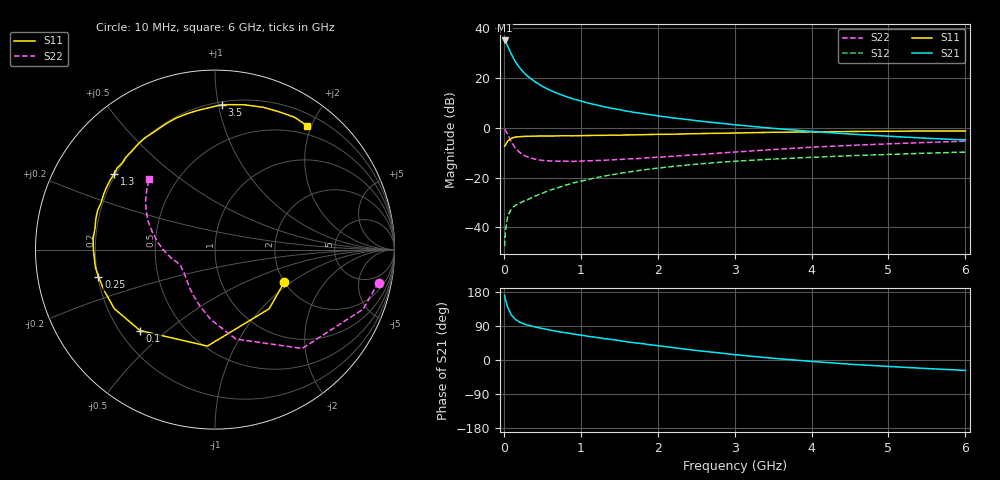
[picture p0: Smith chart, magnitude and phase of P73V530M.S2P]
! SIEMENS Small Signal Semiconductors
! BFP196
! Si NPN RF Bipolar Junction Transistor in SOT143
! VCE = 3.5 V  IC = 30 mA
! Common Emitter S-Parameters:  May  1996
# GHz  S  MA  R  50
!  f  S11  S21  S12  S22
! GHz  MAG  ANG  MAG  ANG  MAG  ANG  MAG  ANG
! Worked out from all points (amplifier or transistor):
!   36 points, 10 MHz to 6 GHz, reference 50 ohm
!   highest |S21| = 35.0 dB at 10 MHz (marker M1)
!   |S21| within 3 dB of that: start of sweep to 61.52 MHz
!   unconditionally stable (mu >= 1): 558.3 MHz to 3.966 GHz
!   at 250 MHz: K = 0.72, MSG = 26.0 dB, |S12| = -29.6 dB
!   at 1.4 GHz: K = 1.09, MAG = 11.5 dB, |S12| = -18.9 dB
!   at 6 GHz: K = 0.98, MSG = 2.4 dB, |S12| = -9.8 dB
!   lowest NFmin = 1.40 dB at 500 MHz
!   S11 on the Smith chart (normalised r, x): 10 MHz: 1.99, -0.89; 100 MHz: 0.28, -0.41; 250 MHz: 0.20, -0.11; 1.3 GHz: 0.19, +0.32; 3.5 GHz: 0.22, +1.03; 6 GHz: 0.37, +1.94
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0.01  0.4262 -25.4  56.22 170.6  0.0042 86.6  0.9293 -11.4
0.02  0.447 -47.5  53.38 160.6  0.0084 73.7  0.8897 -21.9
0.05  0.5392 -94.5  43.61 138.9  0.0169 58.6  0.7343 -48.6
0.1  0.6146 -132.8  29.32 118.2  0.0239 46.8  0.5121 -76.8
0.15  0.6505 -149.6  21.11 107.3  0.0277 44.2  0.3912 -93.3
0.2  0.6585 -159.8  16.38 100.6  0.0301 45.0  0.3256 -105.0
0.25  0.6666 -166.9  13.21 96.1  0.0332 47.1  0.2853 -114.4
0.3  0.6735 -171.5  11.12 92.7  0.0355 48.8  0.2625 -121.1
0.4  0.6771 -179.6  8.451 87.5  0.0421 52.2  0.2346 -131.5
0.5  0.6814 175.2  6.768 83.2  0.0485 54.5  0.2206 -138.9
0.6  0.6791 169.9  5.652 79.1  0.0559 56.3  0.2153 -144.1
0.7  0.6857 165.5  4.864 75.1  0.0622 57.2  0.2129 -148.0
0.9  0.6863 157.6  3.785 68.8  0.0776 57.4  0.211 -153.9
1.1  0.697 150.2  3.116 62.5  0.0918 56.8  0.2166 -157.7
1.3  0.7018 143.3  2.64 56.6  0.1066 55.3  0.2223 -161.3
1.7  0.7176 130.8  2.025 45.4  0.1344 51.1  0.2388 -167.3
2.2  0.7389 116.9  1.57 32.8  0.1674 44.7  0.2666 -174.4
3  0.7815 97.1  1.146 14.1  0.2125 33.9  0.3242 172.1
3.5  0.8086 87.2  0.97 4.6  0.2346 27.4  0.3644 164.0
4.5  0.8375 71.1  0.746 -11.1  0.2738 15.6  0.4414 150.3
5.5  0.8606 58.9  0.613 -22.5  0.3081 4.9  0.5062 138.7
6  0.8597 53.2  0.568 -27.5  0.3244 -0.8  0.5361 133.1
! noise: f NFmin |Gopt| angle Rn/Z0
0.5  1.4  0.4  -173  0.08
0.9  1.6  0.5  -166  0.08
1.5  2.4  0.61  -150  0.14
2  2.9  0.71  -129  0.2
